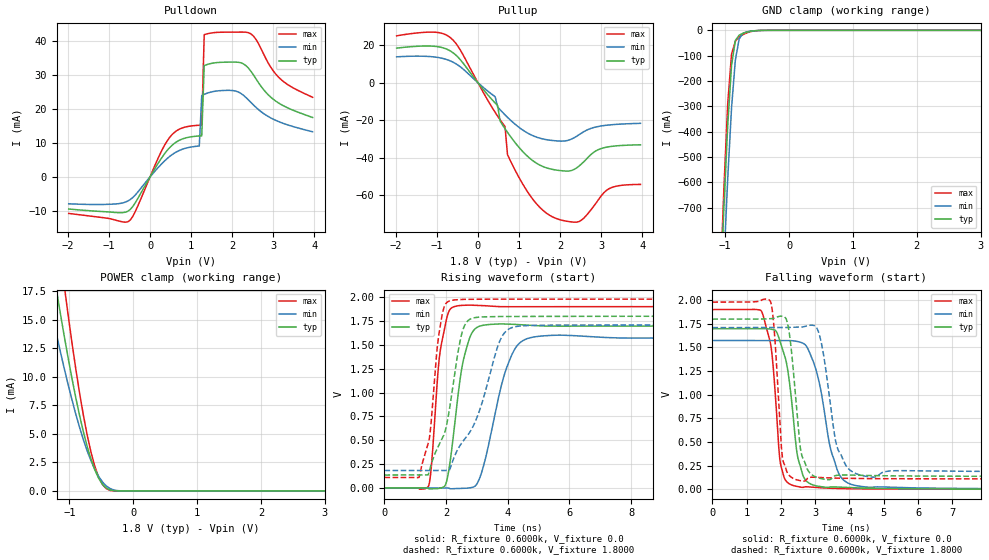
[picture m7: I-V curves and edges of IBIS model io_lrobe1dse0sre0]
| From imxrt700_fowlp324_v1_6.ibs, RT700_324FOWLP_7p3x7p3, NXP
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[Model] io_lrobe1dse0sre0
|   Model io_lrobe1dse0sre0
| This model was characterised for following simulation conditions:
| External (pad) voltage:
|   - Typ: 1.8V,   - Min: 1.71V,   - Max: 1.98V
| Library cells for typ/min/max conditions are connected as defined below:
|  PAD_IO - External Pad
|  ipp_do - Core Input
|  ipp_obe - Output Buffer Enable
|  ASRCN3V3[3] - NC
|  ASRCN3V3[4] - NC
|  ASRCP3V3[4] - NC
|  REFAPBIAS3V3 - gnde
|  REFBAMPL3V3 - vdd1v8
|  REFCAMPH3V3 - vdd1v8
|  REFDNBIAS3V3 - vdd1v8
|  REFH3V3 - REFH3V3
|  REFL3V3 - REFL3V3
|  gnde - gnde
|  ipp_dse - gnde
|  ipp_ina235_3v - NC
|  ipp_ina40_3v - NC
|  ipp_ina_mux - NC
|  ipp_ind - NC
|  ipp_ind_1p8v - NC
|  ipp_ind_3v - NC
|  ipp_sre - gnde
|  vdd - vdd
|  vdd1v8 - vdd1v8
|  vdda - vdde3v3
|  vdde3v3 - vdde3v3
| All other pins connected to ground
Model_type I/O
Polarity   Non-Inverting
Enable   Active-High
Vinl =   0.5400V
Vinh =   1.2600V
Vmeas =  0.9000V
Cref =   15.0000pF
Rref =   0.6000k
Vref =   0.0V
C_comp   3.9800pF   3.7960pF   4.1051pF
|C_comp_pullup   0.3209pF   0.4282pF   0.2791pF
|C_comp_pulldown   2.2501pF   2.3236pF   2.0512pF
[Model Spec]
| variable   typ   min   max
Vinh   1.2600V   NA   NA
Vinl   0.5400V   NA   NA
Vref   0.0V   0.0V   0.0V
Cref   15.0000pF   15.0000pF   15.0000pF
Rref   0.6000k   0.6000k   0.6000k
[Receiver Thresholds]
Vcross_high  =   0.0V
Vcross_low  =   0.0V
Vdiff_ac  =   0.0V
Vdiff_dc  =   0.0V
Tdiffslew_ac  =   0.0S
[Temperature Range]   25.0000   0.1250k   -40.0000
[Voltage Range]   1.8000V   1.7100V   1.9800V
[Pullup Reference]   1.8000V   1.7100V   1.9800V
[Pulldown Reference]   0.0V   0.0V   0.0V
[POWER Clamp Reference]   1.8000V   1.7100V   1.9800V
[GND Clamp Reference]   0.0V   0.0V   0.0V
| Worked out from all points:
|   slope of the pulldown table from 0 to 0.27 V, typ, clamps not added: 50.4 ohm
|   slope of the pullup table from 0 to 0.27 V, typ, clamps not added: 37.3 ohm
|   GND clamp passes 1 mA (typ) near -0.50 V on its own axis
|   POWER clamp passes 1 mA (typ) near -0.53 V on its own axis
|   rising waveform, R_fixture 0.6000k, V_fixture 0.0: 20-80 % time 416ps typ, 681ps min, 294ps max; typ from 0 V to 1.7 V
|   rising waveform, R_fixture 0.6000k, V_fixture 1.8000: 20-80 % time 613ps typ, 1.05ns min, 328ps max; typ from 0.135 V to 1.8 V
|   falling waveform, R_fixture 0.6000k, V_fixture 0.0: 20-80 % time 341ps typ, 519ps min, 244ps max; typ from 1.7 V to 0 V
|   falling waveform, R_fixture 0.6000k, V_fixture 1.8000: 20-80 % time 249ps typ, 358ps min, 185ps max; typ from 1.8 V to 0.135 V
[Pulldown]
|Voltage   I(typ)   I(min)   I(max)
-1.98V    -9.436mA   -7.895mA   -10.73mA
-480mV    -9.541mA   -6.639mA   -12.66mA
480mV     8.648mA    6.047mA    11.65mA
780mV     11.14mA    8.115mA    14.39mA
1.2V      12.06mA    9.106mA    15.21mA
1.26V     12.11mA    23.95mA    15.25mA
1.32V     32.75mA    24.3mA     41.84mA
2.04V     33.78mA    25.37mA    42.6mA
2.46V     31.05mA    21.89mA    42.07mA
2.82V     24.92mA    18.22mA    34.85mA
3.12V     21.84mA    16.35mA    29.49mA
3.96V     17.49mA    13.29mA    23.43mA
[Pullup]
|Voltage   I(typ)   I(min)   I(max)
-1.98V    18.49mA    13.82mA    25.02mA
-960mV    19.18mA    13.43mA    26.78mA
-540mV    14.81mA    10.16mA    21.1mA
480mV     -12.23mA   -12.98mA   -17.88mA
540mV     -20.55mA   -14.43mA   -19.82mA
660mV     -24.59mA   -17.2mA    -23.43mA
720mV     -26.52mA   -18.51mA   -38.45mA
960mV     -33.51mA   -23.18mA   -49.04mA
1.74V     -45.96mA   -30.69mA   -70.78mA
2.46V     -44.61mA   -27.85mA   -74.24mA
3.18V     -34.28mA   -22.63mA   -56.83mA
3.96V     -33.2mA    -21.72mA   -54.36mA
[GND_clamp]
|Voltage   I(typ)   I(min)   I(max)
-1.98V    -7.543A    -7.6A      -7.897A
-1.08V    -1.077A    -1.286A    -1.025A
-1.02V    -705.3mA   -921.3mA   -628.8mA
-960mV    -377.1mA   -587.4mA   -291.7mA
-900mV    -139.2mA   -307mA     -94.38mA
-840mV    -40.12mA   -117mA     -42.82mA
-780mV    -18.81mA   -33.95mA   -26.13mA
-720mV    -11.86mA   -11.44mA   -16.78mA
-660mV    -7.061mA   -5.737mA   -9.992mA
-540mV    -1.684mA   -1.901mA   -2.15mA
-420mV    -207.1uA   -403.7uA   -160.6uA
3.96V     0A         0A         0A
[POWER_clamp]
|Voltage   I(typ)   I(min)   I(max)
-1.98V    46.79mA    35.95mA    61.44mA
-1.32V    21.78mA    16.85mA    28.96mA
-1.2V     17.57mA    13.71mA    23.37mA
-1.08V    13.59mA    10.75mA    18.03mA
-1.02V    11.71mA    9.354mA    15.49mA
-900mV    8.21mA     6.76mA     10.75mA
-720mV    3.899mA    3.511mA    4.896mA
-600mV    1.839mA    1.889mA    2.143mA
-540mV    1.103mA    1.267mA    1.197mA
-420mV    244.5uA    429.3uA    190.7uA
-180mV    281nA      5.273uA    27.6nA
3.96V     0A         0A         0A
[Ramp]
| variable   typ   min   max
dV/dt_r  1.0188/0.4158n   0.9441/0.6813n   1.1406/0.2937n
dV/dt_f  0.9990/0.2491n   0.9166/0.3581n   1.1224/0.1850n
R_load = 0.6000k
[Rising Waveform]
R_fixture= 0.6000k
V_fixture= 0.0
V_fixture_min= 0.0
V_fixture_max= 0.0
|time   V(typ)   V(min)   V(max)
0s        119.2nV    3.183uV    128.2nV
1.427ns   -8.636mV   -705.6uV   17.75mV
1.521ns   -9.714mV   -1.016mV   223.1mV
1.823ns   -1.68mV    -1.054mV   1.467V
2.058ns   131.1mV    -630uV     1.824V
2.456ns   1.145V     -6.141mV   1.912V
2.996ns   1.682V     40.95mV    1.915V
4.14ns    1.716V     1.402V     1.9V
5.156ns   1.698V     1.594V     1.9V
60ns      1.698V     1.573V     1.901V
[Rising Waveform]
R_fixture= 0.6000k
V_fixture= 1.8000
V_fixture_min= 1.7100
V_fixture_max= 1.9800
|time   V(typ)   V(min)   V(max)
0s        135mV      182.4mV    109.3mV
1.127ns   134.2mV    182.3mV    115.3mV
1.466ns   191.5mV    181.6mV    540.4mV
1.707ns   409mV      181.6mV    1.457V
1.882ns   523.1mV    182mV      1.832V
2.276ns   1.195V     334.6mV    1.971V
2.722ns   1.757V     562.2mV    1.977V
3.792ns   1.797V     1.576V     1.979V
4.479ns   1.798V     1.699V     1.979V
60ns      1.8V       1.71V      1.98V
[Falling Waveform]
R_fixture= 0.6000k
V_fixture= 0.0
V_fixture_min= 0.0
V_fixture_max= 0.0
|time   V(typ)   V(min)   V(max)
0s        1.698V     1.573V     1.901V
1.433ns   1.699V     1.573V     1.883V
1.715ns   1.693V     1.574V     1.502V
1.873ns   1.664V     1.573V     811.5mV
2.079ns   1.448V     1.574V     138.9mV
2.613ns   178.1mV    1.549V     19.15mV
3.041ns   34.43mV    1.243V     17.29mV
3.684ns   21.55mV    168.5mV    6.861mV
4.581ns   9.597mV    19.54mV    2.338mV
60ns      7.275uV    14.93uV    3.599uV
[Falling Waveform]
R_fixture= 0.6000k
V_fixture= 1.8000
V_fixture_min= 1.7100
V_fixture_max= 1.9800
|time   V(typ)   V(min)   V(max)
0s        1.8V       1.71V      1.98V
1.69ns    1.804V     1.71V      1.99V
1.817ns   1.813V     1.709V     1.631V
2.061ns   1.828V     1.71V      301.6mV
2.252ns   1.634V     1.712V     142.3mV
2.657ns   314.9mV    1.719V     84.63mV
3.125ns   115.7mV    1.632V     123.8mV
3.672ns   148.3mV    413.2mV    116.3mV
4.643ns   144mV      128.1mV    111.4mV
60ns      135mV      182.4mV    109.3mV
